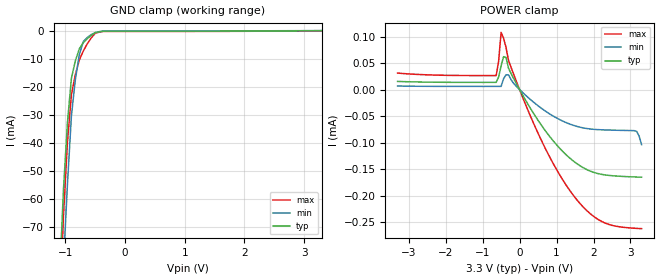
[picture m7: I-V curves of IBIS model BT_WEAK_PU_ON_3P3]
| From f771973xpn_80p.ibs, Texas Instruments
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|   Model Cell BT_WEAK_PU_ON_3P3
|BT_WEAK_PU_ON_3P3
[Model]   BT_WEAK_PU_ON_3P3
Model_type   Input
Polarity   Non-Inverting
Vinl =  0.8
Vinh =  2
C_comp   3.98845p   2.03906p   4.55356p
[Model Spec]
Vinl   0.8   0.8   0.8
Vinh   2   2   2
[Temperature Range]   25   155   -40
[Voltage Range]   3.3   2.97   3.63
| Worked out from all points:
|   GND clamp passes 1 mA (typ) near -0.52 V on its own axis
| Nom Voltages:
|   BIASFET=3.3, VDD=1.2, VDDS=3.3, VSS=0
| Min Voltages:
|   BIASFET=2.97, VDD=1.08, VDDS=2.97, VSS=0
| Max Voltages:
|   BIASFET=3.63, VDD=1.32, VDDS=3.63, VSS=0
[POWER_clamp]
|   voltage   I(typ)   I(min)   I(max)
-3.3V     15.41uA    6.707uA    31.17uA
-633.3mV  13.58uA    5.99uA     26.47uA
-566.7mV  23.9uA     5.99uA     53.64uA
-500mV    44.55uA    5.991uA    108uA
-433.3mV  62.17uA    20.59uA    97.14uA
-366.7mV  60.8uA     27.84uA    79.56uA
-300mV    40.42uA    27.75uA    55.24uA
300mV     -36.17uA   -19.17uA   -51.11uA
1.367V    -129.8uA   -65.26uA   -191.2uA
2.233V    -160.2uA   -75.95uA   -249.4uA
3.167V    -165.1uA   -78.78uA   -262uA
3.3V      -165.4uA   -103.9uA   -262.6uA
[GND_clamp]
|   voltage   I(typ)   I(min)   I(max)
-3.3V     -1.746A    -1.481A    -2.454A
-1.1V     -88.7mA    -114.8mA   -101.4mA
-1.033V   -56.65mA   -82.94mA   -65.98mA
-966.7mV  -32.73mA   -54.79mA   -39.78mA
-900mV    -16.96mA   -30.37mA   -22.8mA
-833.3mV  -10.67mA   -17.32mA   -15.61mA
-766.7mV  -6.426mA   -8.477mA   -10.41mA
-700mV    -4.239mA   -3.852mA   -7.218mA
-566.7mV  -1.643mA   -1.374mA   -2.547mA
-500mV    -691.9uA   -701.6uA   -932.5uA
-366.7mV  -197.1uA   -166.8uA   -293.7uA
3.3V      1.399nA    35.22uA    -55.96uA
